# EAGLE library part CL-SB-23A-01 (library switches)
SWITCH SLIDE DP3T 0.2A JLEAD
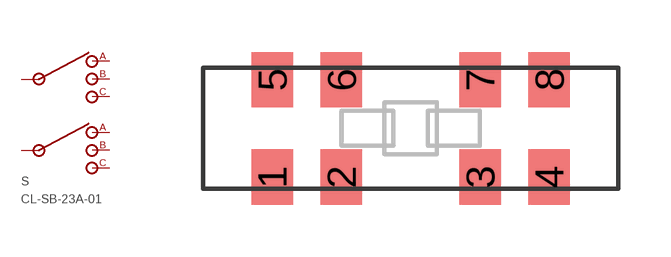
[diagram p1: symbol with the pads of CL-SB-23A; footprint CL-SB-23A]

Designator prefix S

## CL-SB-23A-01 (DIGIKEY: 563-1350-1-ND)  [CL-SB-23A]
1  1
2  2
3  3
4  4
5  5
6  6
7  7
8  8

## Footprint CL-SB-23A (pad centres in mm)
smd 1.2 x 1.6: 1 -4,-1.4; 2 -2,-1.4; 3 2,-1.4; 4 4,-1.4; 5 -4,1.4; 6 -2,1.4; 7 2,1.4; 8 4,1.4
